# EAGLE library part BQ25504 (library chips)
TI BQ25504 Ultra Low Power Boost Converter with Battery Management for Energy Harvester Applications
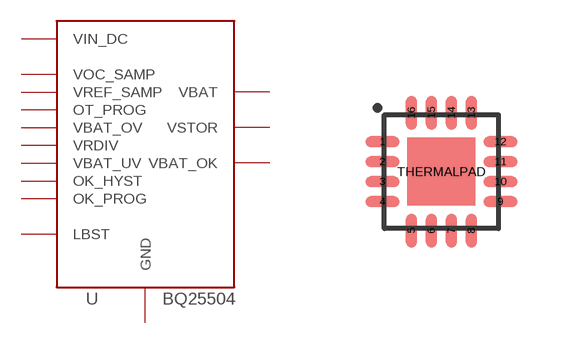
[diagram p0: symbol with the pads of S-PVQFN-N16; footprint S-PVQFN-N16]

Designator prefix U

## BQ25504RGT (DIGIKEY: 296-29741-1-ND)  [S-PVQFN-N16]
1  GND
2  VIN_DC
3  VOC_SAMP
4  VREF_SAMP
5  OT_PROG
6  VBAT_OV
7  VRDIV
8  VBAT_UV
9  OK_HYST
10  OK_PROG
11  VBAT_OK
12  GND
13  GND
14  VBAT
15  VSTOR
16  LBST

## Footprint S-PVQFN-N16 (pad centres in mm)
smd 0.85 x 0.28: 1 -1.475,0.75; 2 -1.475,0.25; 3 -1.475,-0.25; 4 -1.475,-0.75; 9 1.475,-0.75; 10 1.475,-0.25; 11 1.475,0.25; 12 1.475,0.75
smd 0.28 x 0.85: 5 -0.75,-1.475; 6 -0.25,-1.475; 7 0.25,-1.475; 8 0.75,-1.475; 13 0.75,1.475; 14 0.25,1.475; 15 -0.25,1.475; 16 -0.75,1.475
smd 1.7 x 1.7: THERMALPAD 0,0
